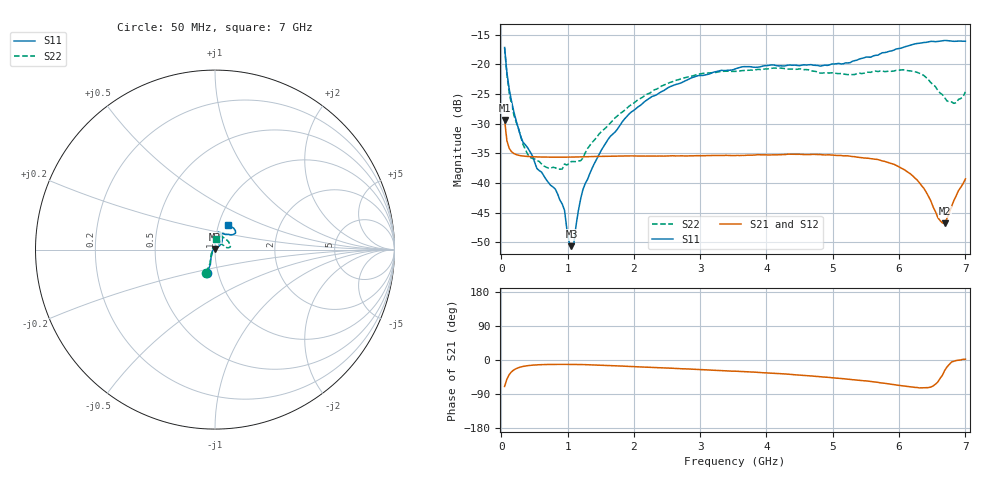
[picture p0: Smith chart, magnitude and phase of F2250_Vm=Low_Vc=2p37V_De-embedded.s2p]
! Integrated Device Technology
! Corporate Headquarters
! 6024 Silver Creek Valley Road
! San Jose, CA 95138  USA
! Phone:  1-408-284-8200
! Toll Free:  1-800-223-1366
! Webpage:  http://www.idt.com/
! Timing and RF Division
! 515 Groton Road, Suite 102
! Westford, MA 01886-6024
! Device:  F2250
! Description: Voltage Variable RF Attenuator
! Frequency:  50.0 -  6000.00 MHz
! Package:  3x3 mm Thin QFN Plastic Package: 16 pin
! Ports:  2 RF, 3 DC
!  Pin  1  = GND
!  Pin  2  = NC
!  Pin  3  = RF1  = Port 1
!  Pin  4  = NC
!  Pin  5  = GND
!  Pin  6  = GND
!  Pin  7  = GND
!  Pin  8  = GND
!  Pin  9  = NC
!  Pin 10  = RF2  = Port 2
!  Pin 11  = NC
!  Pin 12  = GND
!  Pin 13  = GND
!  Pin 14  = VCNTRL
!  Pin 15  = VDD
!  Pin 16  = VMODE
! Vcntrl:  2.370 Volts
! Vmode:  +0.000 Volts
! Vdd:  +3.30  Volts
! Current:  1.177 mA
! Data:  The device was measured on a the F2250 evaluation board which has
!  individual transmission lines to the RF pins.  Data was collected
!  using a calibrated network analyzer.  The evaluation board was
!  de-embedded using a TRL calibration technique.
!  The reference plane is the edge of the package pin.
! Misc:  SN 10
!  Action Tracker AT0258
! Date Measured:  2014-11-26
! Date:  2015-10-15  MJV
! Note:
!  Integrated Device Technology supplies this data as a sample of measured
!  data at the package pin for this product.  Your particular data for this
!  product may vary.
!  Data was taken at 25 degrees C.
!  Integrated Device Technology reserves the right to change this data at anytime.
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# GHz S dB R 50
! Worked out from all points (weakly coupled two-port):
!   201 points, 50 MHz to 7 GHz, reference 50 ohm
!   highest |S21| = -29.41 dB at 50 MHz (marker M1); lowest = -46.8 dB at 6.687 GHz (marker M2)
!   lowest |S11| = -50.7 dB at 1.058 GHz (marker M3), VSWR 1.01, Z = 49.8 + j0.244 ohm
!   |S11| at or under -10 dB: start of sweep to end of sweep
!   |S22| runs from -37.7 to -17.3 dB; largest |S21 - S12| = 6.1e-05
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0.05  -17.18 -108.6  -29.41 -69.8  -29.41 -69.8  -17.29 -110.9
0.08475  -21.44 -107.4  -32.91 -50.3  -32.91 -50.3  -21.77 -110.0
0.15425  -26.23 -116.6  -34.75 -31.1  -34.75 -31.1  -26.85 -122.1
0.29325  -32.20 -127.8  -35.42 -18.5  -35.42 -18.4  -32.19 -137.1
0.3975  -34.08 -141.8  -35.55 -15.0  -35.55 -15.0  -35.18 -160.2
0.5365  -37.56 -155.7  -35.63 -12.8  -35.63 -12.8  -36.20 178.3
0.91875  -43.55 158.0  -35.67 -11.5  -35.68 -11.5  -37.67 132.8
0.9535  -44.61 169.6  -35.67 -11.5  -35.67 -11.5  -36.82 130.6
1.023  -50.01 143.9  -35.66 -11.6  -35.66 -11.6  -36.73 115.0
1.05775  -50.67 123.2  -35.66 -11.6  -35.66 -11.6  -36.40 109.9
1.0925  -50.39 89.6  -35.64 -11.7  -35.65 -11.7  -36.40 105.2
1.162  -44.72 56.7  -35.62 -11.9  -35.63 -11.9  -36.31 94.5
1.2315  -41.12 44.3  -35.60 -12.1  -35.60 -12.1  -35.83 84.9
1.6485  -32.11 41.9  -35.51 -14.6  -35.51 -14.6  -29.87 64.1
2.37825  -24.88 47.3  -35.47 -20.3  -35.47 -20.3  -23.99 56.6
3.525  -20.80 72.4  -35.40 -29.5  -35.40 -29.6  -21.21 74.7
4.7065  -20.17 72.3  -35.19 -42.5  -35.20 -42.6  -21.17 72.2
5.85325  -17.81 40.5  -36.63 -63.2  -36.63 -63.3  -21.14 22.8
6.27025  -16.50 40.1  -39.49 -72.6  -39.49 -72.6  -21.36 9.5
6.68725  -15.99 48.8  -46.84 -27.8  -46.80 -27.4  -25.66 28.3
6.861  -16.13 55.1  -42.18 -1.4  -42.13 -1.3  -26.50 58.0
7  -16.13 63.2  -39.34 1.8  -39.30 1.7  -24.65 83.2
